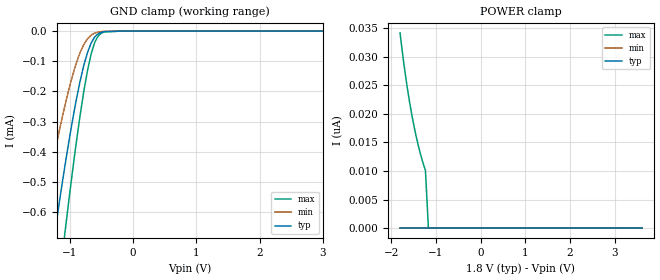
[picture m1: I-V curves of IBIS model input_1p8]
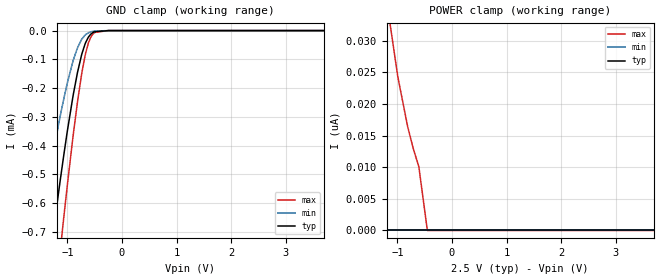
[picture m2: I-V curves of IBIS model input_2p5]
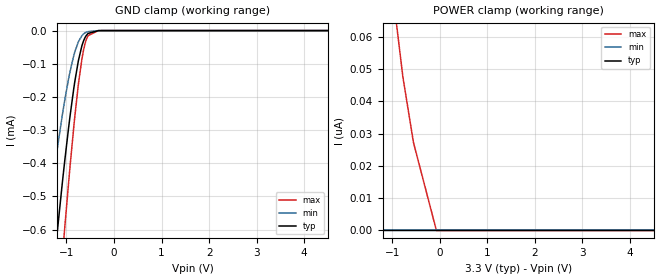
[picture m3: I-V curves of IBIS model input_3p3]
|Texas Instruments Incorporated
| Single Power Supply Single Buffer GATE with 3-State Output CMOS Logic
| Level Shifter
| Marketing part#   Digital Voltage Range   Package-type   #pins
| SN74LV1T126DBV   1.6V-5.5V   SOT-23   5
| SN74LV1T126DCK   1.6V-5.5V   SC70   5
[IBIS Ver]   4.1
[File name]   sn74lv1t126.ibs
[File Rev]   2.0
[Date]   12/27/2013
[Source]
| Texas Instruments Incorporated.
| Analog-eLab Design Center, HPA
| 12500 TI Blvd
| Dallas, TX -75243
[Notes]   Revision History:
| Rev 1.0: 11/08/2013
| - Initial version of the model based on parent device AHCT1G126, 5V.
| Rev 2.0: 12/27/2013
| - All new models for all voltage ranges.
| - Model generated from simulations in TISPICE
| - Model matched to SPICE simulation
| - C_comp although listed in numerical order of value are
|   obtained from varying PVT conditions. For PVT conditions for
|   each specific value refer the buffer description under
|   respective [Model]. IBIS model user is responsible for using
|   appropriate C_comp to simulate for Signal Integrity.
[Disclaimer]
| This model is designed as an aid for customers of Texas Instruments.
| TI and its licensors and suppliers make no warranties, either expressed
| or implied, with respect to this  model, including the warranties of
| merchantability or fitness for a particular purpose. The model is
| provided solely on an "as is" basis. The entire risk as to its quality
| and performance is with the customer.
[Copyright]
(C) Copyright 2013 Texas Instruments Incorporated.All rights reserved.
|   SN74LV1T126DBV
[Component]   SN74LV1T126DBV
[Manufacturer]   TI
[Package]   |5 SOT-23  -  DBV package
|   typ   min   max
R_pkg   0.06117   0.04901   0.06930
L_pkg   1.81421nH   1.46720nH   2.03493nH
C_pkg   0.26116pF   0.24889pF   0.27839pF
[Pin]  signal_name   model_name   R_pin   L_pin   C_pin
1   OE   INPUT   0.06930   2.03493nH  0.27839pF
2   A   INPUT   0.04901   1.46720nH  0.25621pF
3   GND   GND   0.06725   2.43392nH  0.39450pF
4   Y   TRISTATE   0.06519   1.94049nH  0.24889pF
5   VCC   POWER   0.06569   1.95000nH  0.24966pF
|   SN74LV1T126DCK
[Component]   SN74LV1T126DCK
[Manufacturer]   TI
[Package]   |5 SC70   -  DCK package
|   typ   min   max
R_pkg   0.04640   0.04442   0.04813
L_pkg   1.56554nH   1.43808nH   1.64767nH
C_pkg   0.23444pF   0.22838pF   0.23942pF
[Pin]  signal_name   model_name   R_pin   L_pin   C_pin
1   OE   INPUT   0.04813   1.61087nH  0.23942pF
2   A   INPUT   0.04442   1.43808nH  0.23553pF
3   GND   GND   0.04542   1.65485nH  0.26087pF
4   Y   TRISTATE   0.04665   1.64767nH  0.22838pF
5   VCC   POWER   0.04712   1.65572nH  0.22909pF
|   Model Selectors
[Model Selector] INPUT
input_1p8   1.8V  digital input
input_2p5   2.5V  digital input
input_3p3   3.3V  digital input
input_5   5.0V  digital input
[Model Selector] TRISTATE
tristate_1p8   1.8V  digital 3-state
tristate_2p5   2.5V  digital 3-state
tristate_3p3   3.3V  digital 3-state
tristate_5   5.0V  digital 3-state
| Models and submodels in the file (8): input_1p8 (Input), input_2p5 (Input), input_3p3 (Input), input_5 (Input), tristate_1p8 (3-state), tristate_2p5 (3-state), tristate_3p3 (3-state), tristate_5 (3-state)
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|   input_1p8 Model
[Model]   input_1p8
Model_type   Input
Vinl = 0.57
Vinh = 0.95
|   typ   min   max
|   (nom PVT)   (fast PVT)   (slow PVT)
C_comp   5.160e-13   5.160e-13   5.204e-13
[Model spec]
|subparameter
Vinl   0.57   0.57   0.57
Vinh   0.95   0.95   0.99
| Where nom  PVT is Nominal Process, 1.8V, 40C
|   Fast PVT is Strong Process,  1.98V, -40C
|   Slow PVT is Weak Process,   1.62V, 140C
[Voltage Range]   1.8   1.62   1.98
|Junction Temperature
[Temperature Range]   40   140   -40
[Power Clamp Reference]   1.8   1.62   1.98
[GND Clamp Reference]   0   0   0
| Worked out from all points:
|   GND clamp passes 1 mA (typ) near -1.46 V on its own axis
[GND Clamp]
|   Voltage   I(typ)   I(min)   I(max)
-1.8V     -1.557mA   -1.052mA   -2.05mA
-1.498V   -1.063mA   -686uA     -1.452mA
-1.444V   -978.3uA   -624.2uA   -1.347mA
-1.234V   -662.6uA   -397.1uA   -949.8uA
-1.071V   -437.2uA   -240.7uA   -656.2uA
-938.7mV  -273uA     -133.9uA   -433.1uA
-835.2mV  -163.1uA   -69.89uA   -275.3uA
-716.9mV  -68.46uA   -24.53uA   -126.4uA
-658.8mV  -37.89uA   -12.86uA   -72.37uA
-564.5mV  -11.04uA   -3.955uA   -20.29uA
-453.6mV  -1.91uA    -895.5nA   -2.683uA
3.6V      0A         0A         0A
[POWER Clamp]
|   Voltage   I(typ)   I(min)   I(max)
-1.8V     0A         0A         34.15nA
-1.731V   0A         0A         29.7nA
-1.695V   0A         0A         27.61nA
-1.624V   0A         0A         23.82nA
-1.549V   0A         0A         20.31nA
-1.469V   0A         0A         17.12nA
-1.388V   0A         0A         14.32nA
-1.303V   0A         0A         11.83nA
-1.233V   0A         0A         10.09nA
-1.166V   0A         0A         0A
3.6V      0A         0A         0A
|   input_2p5 Model
[Model]   input_2p5
Model_type   Input
Vinl = 0.75
Vinh = 1.145
|   typ   min   max
|   (nom PVT)   (fast PVT)   (slow PVT)
 C_comp   5.160e-13   5.160e-13   5.189e-13
[Model spec]
|subparameter
Vinl   0.75   0.75   0.75
Vinh   1.145   1.145   1.22
| Where nom  PVT is Nominal Process, 2.5V, 40C
|   Fast PVT is Strong Process,  2.75V, -40C
|   Slow PVT is Weak Process,   2.25V, 140C
[Voltage Range]   2.5   2.25   2.75
|Junction Temperature
[Temperature Range]   40   140   -40
[Power Clamp Reference]   2.5   2.25   2.75
[GND Clamp Reference]   0   0   0
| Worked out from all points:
|   GND clamp passes 1 mA (typ) near -1.46 V on its own axis
[GND Clamp]
|   Voltage   I(typ)   I(min)   I(max)
-2.5V     -2.79mA    -1.992mA   -3.485mA
-1.502V   -1.071mA   -691.1uA   -1.46mA
-1.282V   -734.1uA   -447.2uA   -1.04mA
-1.197V   -611.6uA   -360.5uA   -883.2uA
-1.133V   -521.2uA   -297.4uA   -765.8uA
-1.067V   -432.9uA   -237.1uA   -649.3uA
-817.5mV  -147.5uA   -61.26uA   -250.9uA
-732.5mV  -79.31uA   -28.83uA   -143.7uA
-615mV    -22.62uA   -7.583uA   -42.86uA
-498mV    -4.049uA   -1.643uA   -6.405uA
-250mV    -56.13nA   -52.02nA   -34.32nA
5V        0A         0A         0A
[POWER Clamp]
|   Voltage   I(typ)   I(min)   I(max)
-2.5V     0A         0A         290nA
-1.15V    0A         0A         33.5nA
-990.2mV  0A         0A         24.16nA
-811.5mV  0A         0A         16.37nA
-712.5mV  0A         0A         13.02nA
-607.8mV  0A         0A         10.09nA
-451.2mV  0A         0A         0A
5V        0A         0A         0A
|   input_3p3 Model
[Model]   input_3p3
Model_type   Input
Vinl = 0.8
Vinh = 1.37
|   typ   min   max
|   (nom PVT)   (fast PVT)   (slow PVT)
C_comp   5.175e-13   5.160e-13   5.189e-13
[Model spec]
|subparameter
Vinl   0.8   0.8   0.8
Vinh   1.37   1.37   1.47
| Where nom  PVT is Nominal Process, 3.3V, 40C
|   Fast PVT is Strong Process,  3.6V, -40C
|   Slow PVT is Weak Process,   3V, 140C
[Voltage Range]   3.3   3   3.6
|Junction Temperature
[Temperature Range]   40   140   -40
[Power Clamp Reference]   3.3   3   3.6
[GND Clamp Reference]   0   0   0
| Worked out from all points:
|   GND clamp passes 1 mA (typ) near -1.46 V on its own axis
[GND Clamp]
|   Voltage   I(typ)   I(min)   I(max)
-3.3V     -4.289mA   -3.166mA   -5.17mA
-1.424V   -951.1uA   -603.1uA   -1.311mA
-1.227V   -655.5uA   -390.8uA   -938.5uA
-1.059V   -423.9uA   -230.6uA   -636.3uA
-1.032V   -389.1uA   -207.3uA   -589.6uA
-921mV    -255.1uA   -121.9uA   -405.8uA
-821.7mV  -152.3uA   -63.44uA   -257.1uA
-747mV    -90.2uA    -33.34uA   -160.7uA
-675.6mV  -46.65uA   -15.74uA   -86.97uA
-587.4mV  -15.87uA   -5.369uA   -29.27uA
-330mV    -245nA     -162.6nA   -210.3nA
6.6V      0A         0A         0A
[POWER Clamp]
|   Voltage   I(typ)   I(min)   I(max)
-3.3V     38.26nA    0A         1.19uA
-3.052V   29.28nA    0A         975.1nA
-2.802V   22.11nA    0A         784nA
-2.555V   16.55nA    0A         619.6nA
-2.389V   13.56nA    0A         522.9nA
-2.216V   10.96nA    0A         433.2nA
-2.13V    0A         0A         392.5nA
-1.007V   0A         0A         75.81nA
-776.4mV  0A         0A         47.63nA
-553.2mV  0A         0A         27.25nA
-70.8mV   0A         0A         0A
6.6V      0A         0A         0A
